{attribute 'qualified_only'}
{attribute 'strict'}
TYPE eMyDbState :
(
	aggregation := 0,
	error := 10,
	idle := 20,
	readstruct := 30,
	validationissues := 40,
	validationremaining := 50,
	write := 60,
	createcollection := 70,
	dropcollection := 80,
	updateone := 90,
	updatemany := 100,
	writemany := 110,
	delete := 120,
	deletemany := 130
);
END_TYPE
